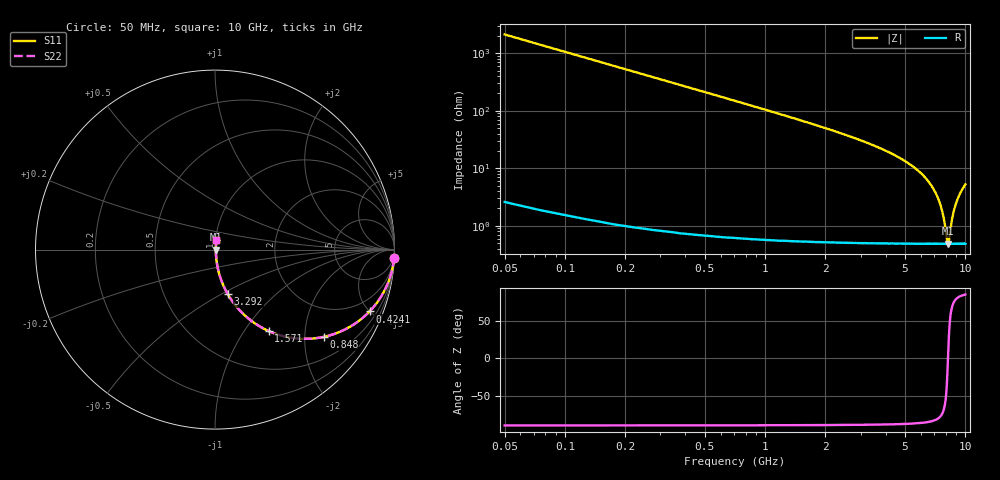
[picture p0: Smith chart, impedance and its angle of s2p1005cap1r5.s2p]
!	AVX	Thin	Film	Operation
!	Date:	March 2012
!	Description: Ultra-Miniature 01005 Size ACCU - P® Thin Film RF / Microwave Capacitor
!	Part Number:  C005YK1R5ABSTR
!	Serial	Measurements
#	MHz	S	db	R	50
!	S11	S21	S12	S22
!	dB	Phase	dB	Phase	dB	Phase	dB	Phase
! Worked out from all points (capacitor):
!   400 points, 50 MHz to 10 GHz, reference 50 ohm
!   read as one part in series: C = 1.5 pF near 99.88 MHz
!   lowest |Z| = 486 mohm at 8.18 GHz (marker M1)
!   series resonance near 8.186 GHz, so ESL is about 250 pH
!   S11 on the Smith chart (normalised r, x): 50 MHz: 1, -42; 424.1 MHz: 1.01, -4.99; 848 MHz: 1.01, -2.48; 1.571 GHz: 1.01, -1.30; 3.292 GHz: 1.01, -0.54; 10 GHz: 1.01, +0.10
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50  -0.01 -2.7  -26.55 87.2  -26.55 87.2  -0.01 -2.7
99.875  -0.04 -5.4  -20.56 84.5  -20.56 84.5  -0.04 -5.4
174.687  -0.12 -9.4  -15.78 80.5  -15.78 80.5  -0.12 -9.4
274.436  -0.29 -14.5  -12.02 75.4  -12.02 75.4  -0.29 -14.5
424.06  -0.66 -21.8  -8.60 68.0  -8.60 68.0  -0.66 -21.8
847.995  -2.20 -38.8  -4.05 50.9  -4.05 50.9  -2.20 -38.8
1571.178  -5.30 -56.6  -1.56 32.9  -1.56 32.9  -5.30 -56.6
1720.802  -5.92 -59.1  -1.33 30.4  -1.33 30.4  -5.92 -59.1
2394.11  -8.54 -67.3  -0.70 22.0  -0.70 22.0  -8.54 -67.3
3291.855  -11.71 -73.9  -0.35 15.0  -0.35 15.0  -11.71 -73.9
3366.667  -11.97 -74.3  -0.33 14.6  -0.33 14.6  -11.97 -74.3
5037.469  -17.77 -80.4  -0.12 7.4  -0.12 7.4  -17.77 -80.4
6708.271  -25.70 -81.7  -0.05 3.0  -0.05 3.0  -25.70 -81.7
7207.018  -29.55 -79.8  -0.05 1.9  -0.05 1.9  -29.55 -79.8
7581.078  -33.81 -75.2  -0.04 1.1  -0.04 1.1  -33.81 -75.2
7830.451  -38.10 -66.5  -0.04 0.7  -0.04 0.7  -38.10 -66.5
8179.574  -46.30 -2.4  -0.04 0.0  -0.04 0.0  -46.30 -2.4
8354.135  -42.93 47.0  -0.04 -0.3  -0.04 -0.3  -42.93 47.0
8603.509  -37.26 68.6  -0.04 -0.7  -0.04 -0.7  -37.26 68.6
8952.632  -32.53 76.9  -0.04 -1.3  -0.04 -1.3  -32.53 76.9
9401.504  -28.84 80.3  -0.05 -2.1  -0.05 -2.1  -28.84 80.3
10000  -25.66 81.7  -0.05 -3.0  -0.05 -3.0  -25.66 81.7
